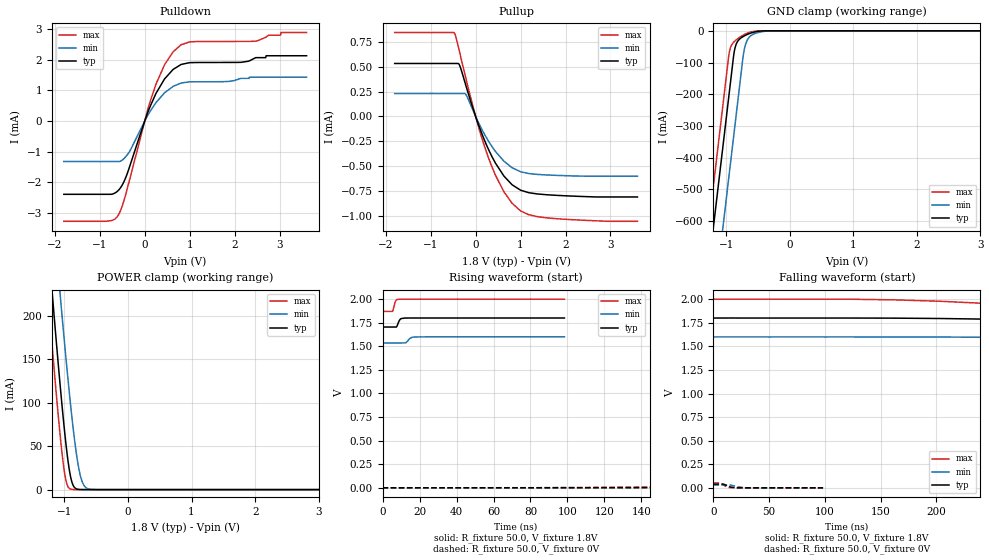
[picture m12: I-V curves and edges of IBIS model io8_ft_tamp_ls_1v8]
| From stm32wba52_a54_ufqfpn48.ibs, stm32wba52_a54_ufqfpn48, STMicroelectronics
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[Model]   io8_ft_tamp_ls_1v8
Model_type I/O
Polarity   Non-Inverting
Enable   Active-Low
| CAP_THRESHOLD on pad IOFT is "UDTCAPC" :
| Rising=30.0% of vddiom   Falling=70.0% of vddiom
| C_comp min and max val. don't necessarily correlate with the min and max pvt
| but are the smallest and greatest pad capacitance found.
| var   typ   min   max
C_comp   6.29519pF  5.93261pF  7.04991pF
|C_comp_pullup   4.08740pF  3.87309pF  4.47657pF
|C_comp_pulldown   2.20780pF  2.05953pF  2.57334pF
Vinl = 800.0mV
Vinh = 1.0V
Vmeas = 900.0mV   | Reference voltage for timing measurements
Cref  = 50.0pF   | Timing specification test load capacitance value
Rref  = 1.0MOhm   | Timing specification test load resistance value
Vref  = 990.0mV   | Timing specification test load voltage
[Model Spec]
| TIME_THRESHOLD on pin ZIV33SW is "CMOS" :
| Rising=50.0% of VDDV33SW   Falling=50.0% of VDDV33SW
Vinl 697.50000mV 636.50000mV 765.50000mV
Vinh 1.08850V 942.50000mV 1.21750V
| variable   typ   min   max
[Temperature Range] 25.0 140.0 -40.0
| variable   typ   min   max
[Voltage Range] 1.8V 1.6V 2.0V
| variable   typ   min   max
[POWER Clamp Reference] 1.8V 1.6V 2.0V
| variable   typ   min   max
[GND Clamp Reference] 0V 0V 0V
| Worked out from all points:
|   slope of the pulldown table from 0 to 0.27 V, typ, clamps not added: 283 ohm
|   slope of the pullup table from 0 to 0.27 V, typ, clamps not added: 855 ohm
|   GND clamp passes 1 mA (typ) near -0.47 V on its own axis
|   POWER clamp passes 1 mA (typ) near -0.81 V on its own axis
|   rising waveform, R_fixture 50.0, V_fixture 1.8V: 20-80 % time 1.34ns typ, 1.94ns min, 1.13ns max; typ from 1.7 V to 1.8 V
|   falling waveform, R_fixture 50.0, V_fixture 1.8V: 20-80 % time 226ns typ, 328ns min, 168ns max; typ from 1.8 V to 1.7 V
[POWER Clamp]
-1.8V     792.8mA    876.2mA    731mA
-1.26V    287mA      389.3mA    225.1mA
-1.19V    224.6mA    328.4mA    163.1mA
-1.06V    114.5mA    218.6mA    57.35mA
-1.02V    83.5mA     186.1mA    30.99mA
-980mV    55.21mA    154.6mA    11.87mA
-910mV    17.39mA    102.5mA    764.6uA
-850mV    3.285mA    62.83mA    47.95uA
-760mV    138.8uA    19.43mA    717.2nA
-700mV    15.66uA    5.838mA    43.61nA
-620mV    848.9nA    820.4uA    1.186nA
3.6V      0A         0A         0A
[GND Clamp]
-1.8V     -1.639A    -1.894A    -1.509A
-1.43V    -1.01A     -1.265A    -879.6mA
-1.24V    -686.9mA   -942.2mA   -556.6mA
-1.05V    -363.9mA   -619.2mA   -233.6mA
-950mV    -193.9mA   -449.2mA   -67.62mA
-870mV    -63.28mA   -313.2mA   -33.62mA
-820mV    -33.62mA   -228.2mA   -25.22mA
-730mV    -17.72mA   -77.21mA   -13.43mA
-690mV    -13.46mA   -40.36mA   -9.392mA
-630mV    -8.329mA   -18.75mA   -4.815mA
-370mV    -86.03uA   -1.078mA   -3.689uA
3.6V      2.71nA     3.15uA     1.142nA
| variable   typ   min   max
[Pullup Reference] 1.8V 1.6V 2.0V
| variable   typ   min   max
[Pulldown Reference] 0V 0V 0V
[Pullup]
-1.8V     532.1uA    230uA      843.1uA
-470mV    532.1uA    230uA      838.2uA
-360mV    517.1uA    230uA      654.4uA
-220mV    315.6uA    221.9uA    388.2uA
60mV      -78.01uA   -58.33uA   -97.65uA
300mV     -345.4uA   -258.9uA   -433.5uA
440mV     -469.3uA   -352uA     -590.3uA
630mV     -600.6uA   -451uA     -758.9uA
810mV     -687.5uA   -516.2uA   -873.7uA
1V        -742.5uA   -557.1uA   -950.7uA
1.6V      -789uA     -589.7uA   -1.021mA
3.6V      -810.9uA   -601.4uA   -1.056mA
[Pulldown]
-1.8V     -2.401mA   -1.328mA   -3.284mA
-870mV    -2.401mA   -1.328mA   -3.284mA
-600mV    -2.291mA   -1.328mA   -3.111mA
-490mV    -2.066mA   -1.268mA   -2.736mA
-350mV    -1.554mA   -1.026mA   -1.996mA
60mV      249uA      164.9uA    332.9uA
250mV     902.8uA    602.1uA    1.206mA
440mV     1.374mA    920.4uA    1.837mA
810mV     1.849mA    1.242mA    2.495mA
2.46V     2.065mA    1.432mA    2.609mA
3.03V     2.134mA    1.432mA    2.892mA
3.6V      2.134mA    1.432mA    2.892mA
[Ramp]
dV/dt_r 23.80627mV/247.23859ns 17.67741mV/423.0297ns 31.01874mV/165.1129ns
dV/dt_f 57.45276mV/222.28849ns 38.54806mV/324.05034ns 78.08278mV/166.92676ns
R_load = 50.0
| Removed startup time: 0s 0s 0s  .
| Removed end time: 98.35ns.
[Rising Waveform]
R_fixture   = 50.0
V_fixture   = 1.8V
V_fixture_min = 1.6V
V_fixture_max = 2.0V
0s        1.704V     1.536V     1.87V
5.35ns    1.704V     1.536V     1.87V
7.05ns    1.704V     1.536V     1.978V
7.7ns     1.71V      1.536V     1.994V
8.85ns    1.764V     1.536V     1.999V
10.05ns   1.794V     1.536V     2V
12.45ns   1.799V     1.536V     2V
15.05ns   1.8V       1.586V     2V
18.05ns   1.8V       1.599V     2V
98.35ns   1.8V       1.6V       2V
| Removed startup time: 0s 0s 0s  .
| Removed end time: 1.9984us.
[Falling Waveform]
R_fixture   = 50.0
V_fixture   = 1.8V
V_fixture_min = 1.6V
V_fixture_max = 2.0V
0s        1.8V       1.6V       2V
122.4ns   1.8V       1.6V       1.999V
163.2ns   1.799V     1.6V       1.992V
244.7ns   1.788V     1.597V     1.954V
359.7ns   1.754V     1.586V     1.901V
436.1ns   1.735V     1.576V     1.884V
543.2ns   1.718V     1.561V     1.874V
693.4ns   1.709V     1.548V     1.871V
938.1ns   1.705V     1.539V     1.87V
1.998us   1.704V     1.536V     1.87V
| Removed startup time: 0s 0s 0s  .
| Removed end time: 1.9984us.
[Rising Waveform]
R_fixture   = 50.0
V_fixture   = 0V
V_fixture_min = 0V
V_fixture_max = 0V
0s        26.35nV    4.279uV    25.49nV
81.55ns   49.53uV    21.57uV    437.3uV
122.4ns   781uV      157.7uV    4.622mV
203.9ns   6.258mV    1.478mV    21.2mV
295.6ns   16.36mV    4.82mV     38.27mV
371.3ns   24.49mV    8.178mV    45.6mV
447.5ns   30.37mV    11.87mV    49.12mV
611.8ns   36.83mV    19.32mV    51.29mV
938.1ns   39.43mV    26.95mV    51.73mV
1.998us   39.68mV    29.47mV    51.7mV
| Removed startup time: 0s 0s 0s  .
| Removed end time: 98.4ns.
[Falling Waveform]
R_fixture   = 50.0
V_fixture   = 0V
V_fixture_min = 0V
V_fixture_max = 0V
0s        39.68mV    29.46mV    51.71mV
6.35ns    39.68mV    29.46mV    51.41mV
9.2ns     38.66mV    29.46mV    29.98mV
12.05ns   23.92mV    29.46mV    11.18mV
15.15ns   10.25mV    29.47mV    2.156mV
16.4ns    7.13mV     27.4mV     767.3uV
19.8ns    1.428mV    17mV       194.3uV
22.1ns    356.3uV    11.04mV    83.18uV
31.4ns    17.77uV    676.7uV    3.377uV
98.4ns    2.441uV    6.659uV    4.013uV
